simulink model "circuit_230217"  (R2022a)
settings: Solver=VariableStepAuto  StartTime=-D+0.1e-6  StopTime=34e-6  FixedStep=1e-3  MaxStep=0.1e-6  RelTol=1e-3
model workspace (MATLAB code in the model file):
  sGeo = CreateGeometry()
  sConst = CreateConstants()
libraries: fl_lib x19, nesl_utility x4, ee_lib x2

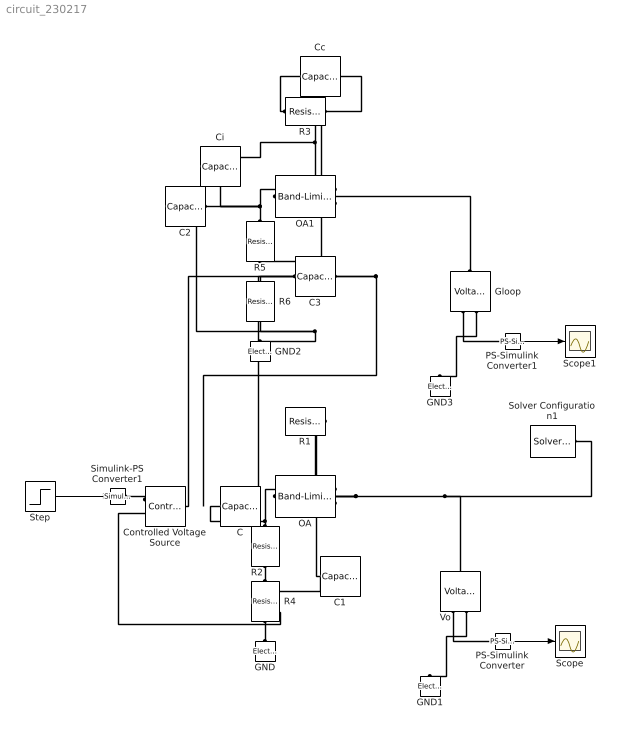
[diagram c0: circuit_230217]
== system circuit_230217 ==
  C{,1..3} (4 alike) : fl_lib/Electrical/Electrical Elements/Capacitor  c=3 uF  r=1e-6 Ohm  g=0 1/Ohm  i_specify=off  i_priority=None  i=0 A  i_nominal_specify=off  i_nominal_unit=A  i_nominal_value=1  v_specify=off  v_priority=None  v=0 V  v_nominal_specify=off  v_nominal_unit=V  v_nominal_value=1  vc_specify=off  vc_priority=High  vc=0 V  vc_nominal_specify=off  vc_nominal_unit=V  vc_nominal_value=1
  Cc : fl_lib/Electrical/Electrical Elements/Capacitor  c=4 pF  r=1e-6 Ohm  g=0 1/Ohm  i_specify=off  i_priority=None  i=0 A  i_nominal_specify=off  i_nominal_unit=A  i_nominal_value=1  v_specify=off  v_priority=None  v=0 V  v_nominal_specify=off  v_nominal_unit=V  v_nominal_value=1  vc_specify=off  vc_priority=High  vc=0 V  vc_nominal_specify=off  vc_nominal_unit=V  vc_nominal_value=1
  Ci : fl_lib/Electrical/Electrical Elements/Capacitor  c=4 pF  r=1e-6 Ohm  g=0 1/Ohm  i_specify=off  i_priority=None  i=0 A  i_nominal_specify=off  i_nominal_unit=A  i_nominal_value=1  v_specify=off  v_priority=None  v=0 V  v_nominal_specify=off  v_nominal_unit=V  v_nominal_value=1  vc_specify=off  vc_priority=High  vc=0 V  vc_nominal_specify=off  vc_nominal_unit=V  vc_nominal_value=1
  Controlled Voltage Source : fl_lib/Electrical/Electrical Sources/Controlled Voltage Source
  GND{,1..3} (4 alike) : fl_lib/Electrical/Electrical Elements/Electrical Reference
  Gloop : fl_lib/Electrical/Electrical Sensors/Voltage Sensor
  OA : ee_lib/Integrated Circuits/Band-Limited Op-Amp  A=100000  Rin=1e8 Ohm  Rout=0 Ohm  Vmin=-15 V  Vmax=15 V  Vdotmax=1000000 V/s  f=5 Hz  V0=0 V
  OA1 : ee_lib/Integrated Circuits/Band-Limited Op-Amp  A=100000  Rin=10 GOhm  Rout=0 Ohm  Vmin=-15 V  Vmax=15 V  Vdotmax=1000000 V/s  f=5 Hz  V0=0 V
  PS-Simulink Converter : nesl_utility/PS-Simulink Converter  PhysicalDomain=network_engine_domain  SubClassName=ps_output  LeftPortType=input  RightPortType=output  PseudoPeriodic=off  Frequencies=[]  VectorFormat=1-D array  Unit=inherit  AffineConversion=off
  PS-Simulink Converter1 : nesl_utility/PS-Simulink Converter  PhysicalDomain=network_engine_domain  SubClassName=ps_output  LeftPortType=input  RightPortType=output  PseudoPeriodic=off  Frequencies=[]  VectorFormat=1-D array  Unit=inherit  AffineConversion=off
  R1 : fl_lib/Electrical/Electrical Elements/Resistor  R=200 kOhm  i_specify=off  i_priority=None  i=0 A  i_nominal_specify=off  i_nominal_unit=A  i_nominal_value=1  v_specify=off  v_priority=None  v=0 V  v_nominal_specify=off  v_nominal_unit=V  v_nominal_value=1
  R{2,4..6} (4 alike) : fl_lib/Electrical/Electrical Elements/Resistor  R=100 kOhm  i_specify=off  i_priority=None  i=0 A  i_nominal_specify=off  i_nominal_unit=A  i_nominal_value=1  v_specify=off  v_priority=None  v=0 V  v_nominal_specify=off  v_nominal_unit=V  v_nominal_value=1
  R3 : fl_lib/Electrical/Electrical Elements/Resistor  R=200 kOhm  i_specify=off  i_priority=None  i=0 A  i_nominal_specify=off  i_nominal_unit=A  i_nominal_value=1  v_specify=off  v_priority=None  v=0 V  v_nominal_specify=off  v_nominal_unit=V  v_nominal_value=1
  Scope : Scope
  Scope1 : Scope
  Simulink-PS Converter1 : nesl_utility/Simulink-PS Converter  PhysicalDomain=network_engine_domain  SubClassName=ps_input  LeftPortType=input  RightPortType=output  PseudoPeriodic=off  Frequencies=[]  NoiseDistribution=none  NoiseParameters=[]  Unit=1  AffineConversion=off  FilteringAndDerivatives=provide  SimscapeFilterOrder=1  InputFilterTimeConstant=0.001  UdotUserProvided=0
  Solver Configuration1 : nesl_utility/Solver Configuration  PhysicalDomain=network_engine_domain  SubClassName=solver  LeftPortType=input  RightPortType=generic  Tones=[]  Harmonics=[]  SimulateNoise=off  Profile=off  UseLocalSampling=off  EnableSwitchedLinearOptims=on  FrequencyDomain=off  UseCCode=off  RelTol=0.001  AbsTol=1e-06  MinStep=1e-09  ToWorkspace=off  RevertToSquareIcSolve=off  NumHomotopyIterations=100  PhasorMode=off  PhasorModeNumHarmonics=1  IndexReductionMethod=DerivativeReplacement  DoDC=off  ResidualTolerance=1e-09  UseLocalSolver=off  LocalSolverChoice=NE_BACKWARD_EULER_ADVANCER  LocalSolverSampleTime=0.001  DoFixedCost=off  MaxNonlinIter=3  MaxModeIter=2  ComputeImpulses=off  ImpulseIterations=2  LinearAlgebra=Sparse  LinearAlgebraNumThread=0  EquationFormulation=NE_TIME_EF  DelaysMemoryBudget=1024  AutomaticFiltering=on  FilteringTimeConstant=0.001  PartitionStorageMethod=AS_NEEDED  PartitionMemoryBudget=1024  PartitionMethod=FAST
  Step : Step  SampleTime=0
  Vo : fl_lib/Electrical/Electrical Sensors/Voltage Sensor
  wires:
  Step/1 -> Simulink-PS Converter1/1
  PS-Simulink Converter/1 -> Scope/1
  PS-Simulink Converter1/1 -> Scope1/1
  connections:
  Vo/RConn1 -- PS-Simulink Converter/LConn1
  Solver Configuration1/RConn1 -- Vo/LConn1 -- C1/LConn1 -- R1/LConn1 -- OA/RConn1
  Controlled Voltage Source/RConn1 -- Simulink-PS Converter1/RConn1
  Vo/RConn2 -- GND1/LConn1
  R2/RConn1 -- C/LConn1 -- OA/LConn1
  R1/RConn1 -- OA/LConn2
  R4/RConn1 -- C1/RConn1 -- R2/LConn1
  R4/LConn1 -- Controlled Voltage Source/RConn2 -- GND/LConn1
  C3/RConn1 -- R6/RConn1 -- R5/LConn1
  C2/RConn1 -- GND2/LConn1 -- R6/LConn1
  Gloop/LConn1 -- OA1/RConn1
  R5/RConn1 -- Ci/LConn1 -- C2/LConn1 -- OA1/LConn1
  Gloop/RConn1 -- PS-Simulink Converter1/LConn1
  Gloop/RConn2 -- GND3/LConn1
  R3/RConn1 -- Cc/LConn1 -- Ci/RConn1 -- OA1/LConn2
  C3/LConn1 -- Controlled Voltage Source/LConn1 -- C/RConn1 -- Cc/RConn1 -- R3/LConn1
